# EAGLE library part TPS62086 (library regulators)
Buck Switching Regulator IC Positive Fixed 3.3V 1 Output 3A 7-VFDFN
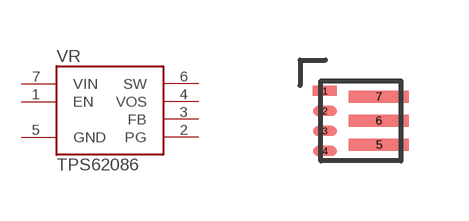
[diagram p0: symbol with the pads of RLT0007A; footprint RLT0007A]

Designator prefix VR

## TPS62086 (DIGIKEY: 296-40831-1-ND)  [RLT0007A]
1  EN
2  PG
3  FB
4  VOS
5  GND
6  SW
7  VIN

## Footprint RLT0007A (pad centres in mm)
smd 0.6 x 0.25: 1 -0.9,0.75; 2 -0.9,0.25; 3 -0.9,-0.25; 4 -0.9,-0.75
smd 1.5 x 0.3: 5 0.45,-0.6; 6 0.45,0; 7 0.45,0.6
